(* Logix 5000 AddOnInstructionDefinition export Banner_R50CMDR_PD_v5; software revision 33.00 *)

TYPE Banner_R50CMDR_PDI_v5 :
STRUCT
   Short_Circuit : BOOL;   // 0=Inactive, 1=Active
   Overcurrent : BOOL;   // 0=Current below limit, 1=Curent above limit
   OverVoltage : BOOL;   // 0=Voltage within Range, 1=Voltage above Range
   UnderVoltage : BOOL;   // 0=Voltage within Range, 1=Voltage below Range
   Block_Temperature : BOOL;   // 0=Temp below limit, 1=Temp above limit
   Aux_Power : BOOL;   // 0=No Aux Power, 1=Aux Power Present
   Pin2_Channel2 : BOOL;   // 0=Inactive, 1=Active
   Pin4_Channel1 : BOOL;   // 0=Inactive, 1=Active
   Pin5_Analog_Value : INT;
END_STRUCT
END_TYPE

TYPE Banner_R50CMDR_PDIO_v5 :
STRUCT
   PDI : Banner_R50CMDR_PDI_v5;
   PDO : Banner_R50CMDR_PDO_v5;
   DTI : SINT[4];
   DTO : SINT[4];
END_STRUCT
END_TYPE

TYPE Banner_R50CMDR_PDO_v5 :
STRUCT
   Motor_Current_Fault_Reset : BOOL;
   Pin2_Channel2_Control : BOOL;
   Pin4_Channel1_Control : BOOL;
   Pin5_Analog_Output_Control : INT;
END_STRUCT
END_TYPE

ADD_ON_INSTRUCTION Banner_R50CMDR_PD_v5   (* revision 5.0 *)
VAR_IN_OUT
   PD : Banner_R50CMDR_PDIO_v5; {required}
END_VAR
VAR_INPUT
   Byte_Sweap : BOOL; {required}
END_VAR
VAR
   TempOut : SINT[4]; {access None}
   TempIn : SINT[4]; {access None}
END_VAR

ROUTINE Logic   (* ladder *)
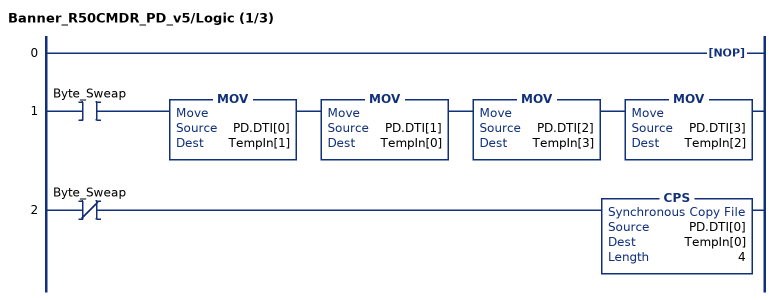
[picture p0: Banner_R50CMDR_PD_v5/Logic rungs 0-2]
   0: NOP();
   1: XIC(Byte_Sweap)MOV(PD.DTI[0],TempIn[1])MOV(PD.DTI[1],TempIn[0])MOV(PD.DTI[2],TempIn[3])MOV(PD.DTI[3],TempIn[2]);
   2: XIO(Byte_Sweap)CPS(PD.DTI[0],TempIn[0],4);
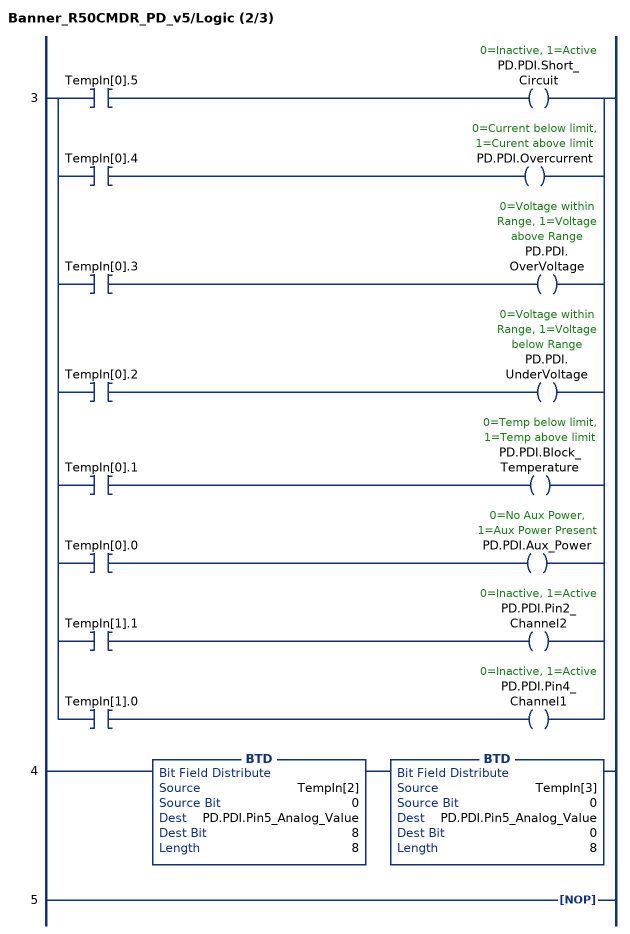
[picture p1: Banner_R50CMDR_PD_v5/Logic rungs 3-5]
   3: [XIC(TempIn[0].5) OTE(PD.PDI.Short_Circuit) ,XIC(TempIn[0].4) OTE(PD.PDI.Overcurrent) ,XIC(TempIn[0].3) OTE(PD.PDI.OverVoltage) ,XIC(TempIn[0].2) OTE(PD.PDI.UnderVoltage) ,XIC(TempIn[0].1) OTE(PD.PDI.Block_Temperature) ,XIC(TempIn[0].0) OTE(PD.PDI.Aux_Power) ,XIC(TempIn[1].1) OTE(PD.PDI.Pin2_Channel2) ,XIC(TempIn[1].0) OTE(PD.PDI.Pin4_Channel1) ];
   4: BTD(TempIn[2],0,PD.PDI.Pin5_Analog_Value,8,8)BTD(TempIn[3],0,PD.PDI.Pin5_Analog_Value,0,8);
   5: NOP();
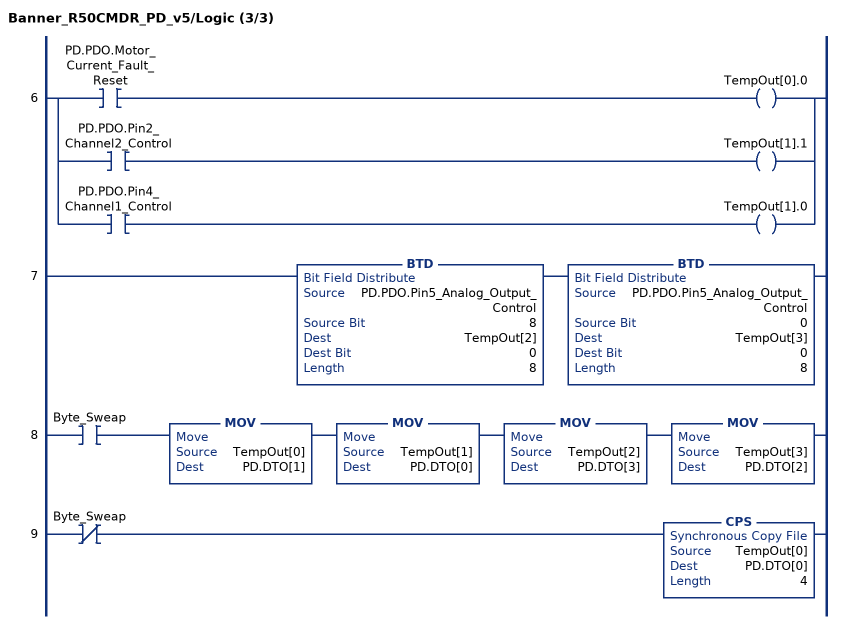
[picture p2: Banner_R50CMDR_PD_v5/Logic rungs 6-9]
   6: [XIC(PD.PDO.Motor_Current_Fault_Reset) OTE(TempOut[0].0) ,XIC(PD.PDO.Pin2_Channel2_Control) OTE(TempOut[1].1) ,XIC(PD.PDO.Pin4_Channel1_Control) OTE(TempOut[1].0) ];
   7: BTD(PD.PDO.Pin5_Analog_Output_Control,8,TempOut[2],0,8)BTD(PD.PDO.Pin5_Analog_Output_Control,0,TempOut[3],0,8);
   8: XIC(Byte_Sweap)MOV(TempOut[0],PD.DTO[1])MOV(TempOut[1],PD.DTO[0])MOV(TempOut[2],PD.DTO[3])MOV(TempOut[3],PD.DTO[2]);
   9: XIO(Byte_Sweap)CPS(TempOut[0],PD.DTO[0],4);
END_ROUTINE
END_ADD_ON_INSTRUCTION
